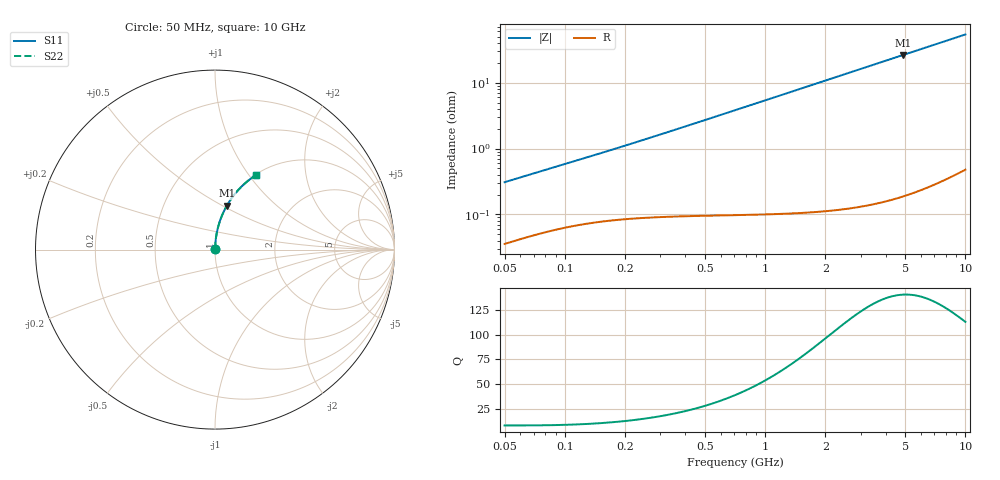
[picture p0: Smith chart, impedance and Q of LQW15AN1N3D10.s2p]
!Murata Part Number: LQW15AN1N3D10
!These Parameters are Measured in Series Mode Connection
!  o--[Z]--o
!Port1  Port2
!  o-------o
!Freq. Start=50[MHz] Stop=10[GHz], 401[Steps]
# Hz S RI R 50
!Freq.(Hz)	S 11(Real)	S 11(Imag)	S 21(Real)	S 21(Imag)	S 12(Real)	S 12(Imag)	S 22(Real)	S 22(Imag)
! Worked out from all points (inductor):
!   401 points, 50 MHz to 10 GHz, reference 50 ohm
!   read as one part in series: L = 958 pH near 51.34 MHz
!   highest Q = 140 at 4.891 GHz (marker M1), where L = 857 pH
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5e7  0.000367 0.00307  0.9996 -0.00307  0.9996 -0.00307  0.000367 0.00307
5.134228e7  0.000376 0.00314  0.9996 -0.00314  0.9996 -0.00314  0.000376 0.00314
1.214486e8  0.000751 0.00691  0.9992 -0.00691  0.9992 -0.00691  0.000751 0.00691
1.880302e8  0.000942 0.0104  0.9991 -0.0104  0.9991 -0.0104  0.000942 0.0104
2.949953e8  0.00117 0.0161  0.9988 -0.0161  0.9988 -0.0161  0.00117 0.0161
4.689809e8  0.00159 0.0253  0.9984 -0.0253  0.9984 -0.0253  0.00159 0.0253
7.071068e8  0.00242 0.038  0.9976 -0.038  0.9976 -0.038  0.00242 0.038
9.094607e8  0.00338 0.0488  0.9966 -0.0488  0.9966 -0.0488  0.00338 0.0488
1.139142e9  0.00475 0.061  0.9952 -0.061  0.9952 -0.061  0.00475 0.061
1.408053e9  0.00674 0.0752  0.9933 -0.0752  0.9933 -0.0752  0.00674 0.0752
1.717543e9  0.00952 0.0915  0.9905 -0.0915  0.9905 -0.0915  0.00952 0.0915
2.179987e9  0.0147 0.1155  0.9853 -0.1155  0.9853 -0.1155  0.0147 0.1155
2.730534e9  0.0223 0.1435  0.9777 -0.1435  0.9777 -0.1435  0.0223 0.1435
3.375117e9  0.0332 0.1753  0.9668 -0.1753  0.9668 -0.1753  0.0332 0.1753
4.171863e9  0.0494 0.2131  0.9506 -0.2131  0.9506 -0.2131  0.0494 0.2131
4.890587e9  0.0663 0.2453  0.9337 -0.2453  0.9337 -0.2453  0.0663 0.2453
5.88704e9  0.0929 0.2868  0.9071 -0.2868  0.9071 -0.2868  0.0929 0.2868
6.993273e9  0.126 0.3281  0.874 -0.3281  0.874 -0.3281  0.126 0.3281
8.198065e9  0.1651 0.3673  0.8349 -0.3673  0.8349 -0.3673  0.1651 0.3673
8.994549e9  0.1921 0.3898  0.8079 -0.3898  0.8079 -0.3898  0.1921 0.3898
9.738562e9  0.2179 0.4085  0.7821 -0.4085  0.7821 -0.4085  0.2179 0.4085
1e10  0.227 0.4145  0.773 -0.4145  0.773 -0.4145  0.227 0.4145
